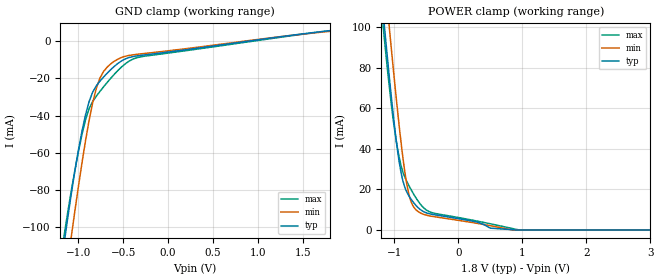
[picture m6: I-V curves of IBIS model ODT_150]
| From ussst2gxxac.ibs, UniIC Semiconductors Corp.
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|   Model ODT_150
[Model]  ODT_150
Model_type Input
Polarity   Non-Inverting
Vinl =   0.70000000V
Vinh =   1.10000000V
C_comp   2.5240pF   2.5060pF   2.5510pF
[Temperature Range]   25.0000   95.0000   0.0
[Voltage Range]   1.8000V   1.7000V   1.9000V
[GND_clamp]
|Voltage   I(typ)   I(min)   I(max)
-1.8V     -351.6mA   -377.6mA   -343.7mA
-1.16V    -109.1mA   -133.9mA   -104.8mA
-1.12V    -95.45mA   -119.6mA   -92.38mA
-1.08V    -82.35mA   -105.4mA   -80.69mA
-1V       -58.63mA   -78.26mA   -59.49mA
-920mV    -39.56mA   -53.42mA   -42.2mA
-880mV    -32.4mA    -42.46mA   -36.28mA
-800mV    -24.01mA   -25.36mA   -29.57mA
-720mV    -19.34mA   -16.36mA   -24.61mA
-600mV    -13.58mA   -10.82mA   -17.82mA
-320mV    -7.76mA    -6.94mA    -8.581mA
1.8V      5.614mA    5.258mA    5.59mA
[POWER_clamp]
|Voltage   I(typ)   I(min)   I(max)
-1.8V     333.7mA    359.4mA    325.6mA
-1.18V    110.3mA    135.8mA    103.5mA
-1.14V    96.79mA    122mA      90.54mA
-1.08V    77.17mA    101.7mA    72.19mA
-1V       53.01mA    75.56mA    51.16mA
-920mV    33.5mA     51.18mA    35.79mA
-800mV    18.62mA    22.27mA    23.84mA
-720mV    14.53mA    12.8mA     19.08mA
-600mV    10.31mA    8.585mA    13.14mA
-400mV    7.694mA    6.698mA    8.483mA
903.9mV   0A         NA         NA
3.6V      0A         0A         0A
